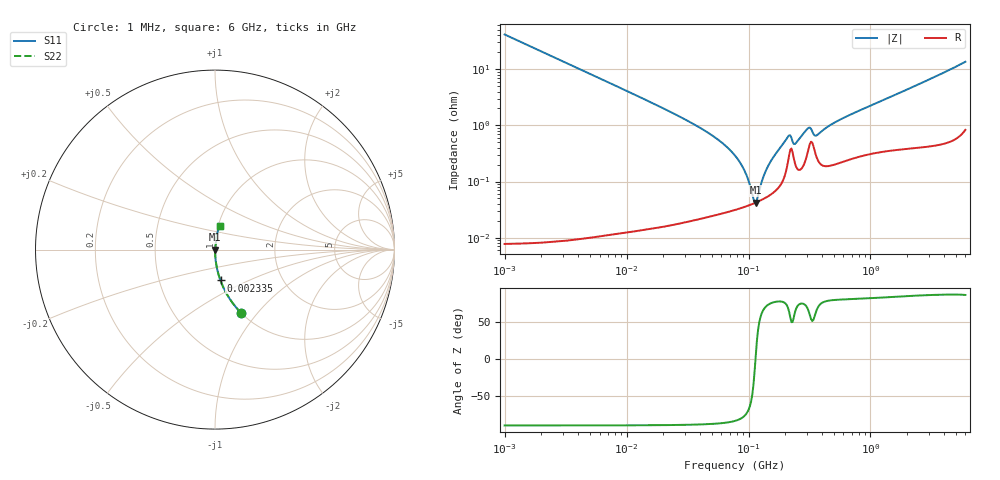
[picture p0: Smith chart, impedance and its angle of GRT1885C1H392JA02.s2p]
!Murata Part Number: GRT1885C1H392JA02
!These Parameters are Measured in Series Mode Connection
!Data Generated on Jun 19, 2026
!  o--ll--o
!Port1  Port2
!  o------o
!Operation Temp=25[degC], DC Bias Voltage=0[V]
!Freq. Start=1000[kHz] Stop=6[GHz] 401[Steps]
# Hz S RI R 50
!Freq.(Hz) S11(Real) S11(Imag) S21(Real) S21(Imag) S12(Real) S12(Imag) S22(Real) S22(Imag)
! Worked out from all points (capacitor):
!   401 points, 1 MHz to 6 GHz, reference 50 ohm
!   read as one part in series: C = 3.84 nF near 1.044 MHz
!   lowest |Z| = 42.2 mohm at 114.6 MHz (marker M1)
!   series resonance near 114.1 MHz, so ESL is about 510 pH
!   S11 on the Smith chart (normalised r, x): 1 MHz: 1.00, -0.83; 2.335 MHz: 1.00, -0.36; 6 GHz: 1.02, +0.27
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1000000  0.1469 -0.3539  0.8531 0.3539  0.8531 0.3539  0.1469 -0.3539
2335446  0.0306 -0.1721  0.9694 0.1721  0.9694 0.1721  0.0306 -0.1721
4293785  0.00931 -0.0956  0.9907 0.0956  0.9907 0.0956  0.00931 -0.0956
1.843659e7  0.000629 -0.0219  0.9994 0.0219  0.9994 0.0219  0.000629 -0.0219
4.697123e7  0.000287 -0.0073  0.9997 0.0073  0.9997 0.0073  0.000287 -0.0073
7.745967e7  0.00032 -0.00288  0.9997 0.00288  0.9997 0.00288  0.00032 -0.00288
9.218041e7  0.000354 -0.00156  0.9996 0.00156  0.9996 0.00156  0.000354 -0.00156
9.83954e7  0.000371 -0.00108  0.9996 0.00108  0.9996 0.00108  0.000371 -0.00108
1.096987e8  0.000405 -0.000286  0.9996 0.000286  0.9996 0.000286  0.000405 -0.000286
1.145757e8  0.000421 3.32e-05  0.9996 -3.32e-05  0.9996 -3.32e-05  0.000421 3.32e-05
1.196694e8  0.000439 0.000354  0.9996 -0.000354  0.9996 -0.000354  0.000439 0.000354
1.334167e8  0.000494 0.00117  0.9995 -0.00117  0.9995 -0.00117  0.000494 0.00117
1.455431e8  0.000553 0.00185  0.9994 -0.00185  0.9994 -0.00185  0.000553 0.00185
2.061188e8  0.00178 0.00556  0.9982 -0.00556  0.9982 -0.00556  0.00178 0.00556
2.152823e8  0.00297 0.0059  0.997 -0.0059  0.997 -0.0059  0.00297 0.0059
2.400133e8  0.00214 0.00412  0.9979 -0.00412  0.9979 -0.00412  0.00214 0.00412
3.048839e8  0.0033 0.00806  0.9967 -0.00806  0.9967 -0.00806  0.0033 0.00806
3.325952e8  0.00495 0.00611  0.995 -0.00611  0.995 -0.00611  0.00495 0.00611
3.628252e8  0.00268 0.00607  0.9973 -0.00607  0.9973 -0.00607  0.00268 0.00607
5.60538e8  0.00229 0.0123  0.9977 -0.0123  0.9977 -0.0123  0.00229 0.0123
1.428092e9  0.00447 0.031  0.9955 -0.031  0.9955 -0.031  0.00447 0.031
6e9  0.0258 0.1309  0.9742 -0.1309  0.9742 -0.1309  0.0258 0.1309
